| Texas Instruments Incorporated
| 24-Bit Analog-to-Digital Converters for Temperature Sensors
| Marketing part#   Voltage Range   Package-type  #pins/pkg drawing
| ADS1146IPW   2.7V - 5.25V   TSSOP   16-pin PW
| ADS1146IPWR   2.7V - 5.25V   TSSOP   16-pin PW
| ADS1147IPW   2.7V - 5.25V   TSSOP   16-pin PW
| ADS1147IPWR   2.7V - 5.25V   TSSOP   16-pin PW
| ADS1148IPW   2.7V - 5.25V   TSSOP   16-pin PW
| ADS1148IPWR   2.7V - 5.25V   TSSOP   16-pin PW
| ADS1246IPW   2.7V - 5.25V   TSSOP   16-pin PW
| ADS1246IPWR   2.7V - 5.25V   TSSOP   16-pin PW
| ADS1247IPW   2.7V - 5.25V   TSSOP   16-pin PW
| ADS1247IPWR   2.7V - 5.25V   TSSOP   16-pin PW
| ADS1248IPW   2.7V - 5.25V   TSSOP   16-pin PW
| ADS1248IPWR   2.7V - 5.25V   TSSOP   16-pin PW
[IBIS ver]   4.0
[File name]   ads1x4x.ibs
[File Rev]   1.0
[Date]   11/28/2009
[Source]   Texas Instruments Incorporated.
   Analog-eLab, HPA
   12500 TI Blvd
   Dallas, TX -75243
   For Support e-mail: elab_ibis@list.ti.com
[Notes]   Revision History
   Rev 1.0: 11/28/2009
   - Initial version of the model
   - Model based on simulations from TIspiceD
   - Model not matched to measurements
   - Ignore warnings related to ccomp, these are
   based on PVT variations as seen in simulations
[Disclaimer] This model is designed as an aid for customers of Texas Instruments.
 TI and its licensors and suppliers make no warranties, either expressed
 or implied, with respect to this  model, including the warranties of
 merchantability or fitness for a particular purpose.
 The model is provided solely on an "as is" basis. The entire risk as to
 its quality and performance is with the customer.
[Copyright] (C)Copyright 2009 Texas Instruments Incorporated.
   All rights reserved.
|   Component ADS1146PW and PWR
[Component]   ADS1146   |16-pin TSSOP PW package
[Manufacturer] TI
[Package]   |16-pin TSSOP PW and PWR package
| variable   typ   min   max
R_pkg  0.0668   0.0264   0.0907
L_pkg  2.1992nH  1.8611nH  2.5678nH
C_pkg  0.2884pF  0.2565pF  0.3511pF
[Pin] signal_name  model_name  R_pin  L_pin C_pin
   1   DVDD   POWER   0.05175  2.54903nH  0.33026pF
   2   DGND   GND   0.07117  2.04833nH  0.27033pF
   3   CLK   CLK   0.06252  1.87476nH  0.26286pF
   4   nRESET   INPUT   0.07117  2.04767nH  0.26971pF
   5   REFP   NC   0.0721   2.06639nH  0.27241pF
   6   REFN   NC   0.08688  2.36796nH  0.28566pF
   7   AINP   NC   0.06167  1.86111nH  0.25647pF
   8   AINN   NC   0.04904  2.50555nH  0.32779pF
   9   AVSS   GND   0.02642  2.28114nH  0.35109pF
   10   AVDD   POWER   0.09072  2.44998nH  0.28608pF
   11   START   INPUT   0.08853  2.40166nH  0.28835pF
   12   nCS   INPUT   0.08017  2.23009nH  0.28047pF
   13   nDRDY   OUTPUT   0.07129  2.04997nH  0.27114pF
   14   DOUT_nDRDY   DOUTPUT   0.06269  1.87807nH  0.26318pF
   15   DIN   INPUT   0.06918  2.00833nH  0.26803pF
   16   SCLK   INPUT   0.05271  2.5678nH   0.33089pF
|   Component ADS1147PW and PWR
[Component]   ADS1147   |20-pin TSSOP PW and PWR package
[Manufacturer] TI
[Package]   |20-pin TSSOP PW package
| variable   typ   min   max
R_pkg   0.0709   0.0340   0.0869
L_pkg   2.3105nH   1.5412nH   3.1530nH
C_pkg   0.3360pF   0.2711pF   0.4455pF
[Pin] signal_name  model_name  R_pin  L_pin C_pin
   1   DVDD   POWER   0.08096  3.14617nH  0.44548pF
   2   DGND   GND   0.07981  2.71014nH  0.38797pF
   3   CLK   CLK   0.06746  1.89158nH  0.27293pF
   4   nRESET   INPUT   0.06568  1.85791nH  0.27112pF
   5   REFP0_GPIO0   GPIO   0.06523  1.84931nH  0.27116pF
   6   REFN0_GPIO1   GPIO   0.07108  1.96470nH  0.27714pF
   7   VREFOUT   NC   0.03398  1.54116nH  0.30506pF
   8   VREFCOM   NC   0.07334  2.00990nH  0.28144pF
   9   AIN0_IEXC   NC   0.08690  2.85399nH  0.39588pF
   10   AIN1_IEXC   NC   0.08052  3.14616nH  0.44428pF
   11   AIN2_IEXC_GPIO2   GPIO   0.08085  3.15303nH  0.44321pF
   12   AIN3_IEXC_GPIO3   GPIO   0.08375  2.79684nH  0.38993pF
   13   AVSS   GND   0.04122  1.78526nH  0.32347pF
   14   AVDD   POWER   0.07359  2.01438nH  0.28108pF
   15   START   INPUT   0.07236  1.98988nH  0.27787pF
   16   nCS   INPUT   0.06814  1.90665nH  0.27392pF
   17   nDRDY   OUTPUT   0.06585  1.86117nH  0.27196pF
   18   DOUT_nDRDY   DOUTPUT   0.06763  1.89484nH  0.27328pF
   19   DIN   INPUT   0.07917  2.69229nH  0.38747pF
   20   SCLK   INPUT   0.08095  3.14559nH  0.44469pF
|   Component ADS1148PW and PWR
[Component]   ADS1148
[Manufacturer]  Texas Instruments Incorporated
[Package]   |28-pin TSSOP PW and PWR package
|   typ   min   max
R_pkg   0.191   0.083   0.299
L_pkg   2.756nH   1.602nH   3.911nH
C_pkg   0.569pF   0.404pF   0.734pF
[Pin] signal_name   model_name   R_pin   L_pin   C_pin
   1   DVDD   POWER   0.25840  3.78183nH   0.72612pF
   2   DGND   GND   0.25457  3.37203nH   0.65437pF
   3   CLK   CLK   0.27139  2.95777nH   0.47887pF
   4   nRESET   INPUT   0.24262  2.60943nH   0.42484pF
   5   REFP0_GPIO0   GPIO   0.23670  2.55749nH   0.43312pF
   6   REFN0_GPIO1   GPIO   0.19699  2.23854nH   0.41962pF
   7   REFP1   NC   0.16925  2.01926nH   0.40844pF
   8   REFN1   NC   0.15863  1.93718nH   0.40408pF
   9   VREFOUT   NC   0.08283  1.60169nH   0.43637pF
   10   VREFCOM   NC   0.18323  2.13341nH   0.41480pF
   11   AIN0_IEXC   NC   0.21768  2.41321nH   0.41552pF
   12   AIN1_IEXC   NC   0.27481  2.99152nH   0.47926pF
   13   AIN4_IEXC_GPIO4   GPIO   0.26374  3.45284nH   0.65872pF
   14   AIN5_IEXC_GPIO5   GPIO   0.26014  3.80161nH   0.72855pF
   15   AIN6_IEXC_GPIO6   GPIO   0.27369  3.91108nH   0.73394pF
   16   AIN7_IEXC_GPIO7   GPIO   0.28429  3.61685nH   0.66751pF
   17   AIN2_IEXC_GPIO2   GPIO   0.29927  3.19031nH   0.48711pF
   18   AIN3_IEXC_GPIO3   GPIO   0.21114  2.36074nH   0.41327pF
   19   IEXC2   NC   0.17260  2.04890nH   0.41119pF
   20   IEXC1   NC   0.15867  1.93751nH   0.40587pF
   21   AVSS   GND   0.08769  1.65289nH   0.44333pF
   22   AVDD   POWER   0.19052  2.18715nH   0.41522pF
   23   START   INPUT   0.19562  2.22790nH   0.41629pF
   24   nCS   INPUT   0.21539  2.38631nH   0.42471pF
   25   nDRDY   OUTPUT   0.24299  2.61259nH   0.42589pF
   26   DOUT_nDRDY   DOUTPUT   0.27156  2.95896nH   0.47947pF
   27   DIN   INPUT   0.25335  3.35997nH   0.65372pF
   28   SCLK   INPUT   0.25851  3.78132nH   0.72511pF
|   Component ADS1246PW and PWR
[Component]   ADS1246   |16-pin TSSOP PW package
[Manufacturer] TI
[Package]   |16-pin TSSOP PW and PWR package
| variable   typ   min   max
R_pkg  0.0668   0.0264   0.0907
L_pkg  2.1992nH  1.8611nH  2.5678nH
C_pkg  0.2884pF  0.2565pF  0.3511pF
[Pin] signal_name  model_name  R_pin  L_pin C_pin
   1   DVDD   POWER   0.05175  2.54903nH  0.33026pF
   2   DGND   GND   0.07117  2.04833nH  0.27033pF
   3   CLK   CLK   0.06252  1.87476nH  0.26286pF
   4   nRESET   INPUT   0.07117  2.04767nH  0.26971pF
   5   REFP   NC   0.0721   2.06639nH  0.27241pF
   6   REFN   NC   0.08688  2.36796nH  0.28566pF
   7   AINP   NC   0.06167  1.86111nH  0.25647pF
   8   AINN   NC   0.04904  2.50555nH  0.32779pF
   9   AVSS   GND   0.02642  2.28114nH  0.35109pF
   10   AVDD   POWER   0.09072  2.44998nH  0.28608pF
   11   START   INPUT   0.08853  2.40166nH  0.28835pF
   12   nCS   INPUT   0.08017  2.23009nH  0.28047pF
   13   nDRDY   OUTPUT   0.07129  2.04997nH  0.27114pF
   14   DOUT_nDRDY   DOUTPUT   0.06269  1.87807nH  0.26318pF
   15   DIN   INPUT   0.06918  2.00833nH  0.26803pF
   16   SCLK   INPUT   0.05271  2.5678nH   0.33089pF
|   Component ADS1247PW and PWR
[Component]   ADS1247   |20-pin TSSOP PW and PWR package
[Manufacturer] TI
[Package]   |20-pin TSSOP PW package
| variable   typ   min   max
R_pkg   0.0709   0.0340   0.0869
L_pkg   2.3105nH   1.5412nH   3.1530nH
C_pkg   0.3360pF   0.2711pF   0.4455pF
[Pin] signal_name  model_name  R_pin  L_pin C_pin
   1   DVDD   POWER   0.08096  3.14617nH  0.44548pF
   2   DGND   GND   0.07981  2.71014nH  0.38797pF
   3   CLK   CLK   0.06746  1.89158nH  0.27293pF
   4   nRESET   INPUT   0.06568  1.85791nH  0.27112pF
   5   REFP0_GPIO0   GPIO   0.06523  1.84931nH  0.27116pF
   6   REFN0_GPIO1   GPIO   0.07108  1.96470nH  0.27714pF
   7   VREFOUT   NC   0.03398  1.54116nH  0.30506pF
   8   VREFCOM   NC   0.07334  2.00990nH  0.28144pF
   9   AIN0_IEXC   NC   0.08690  2.85399nH  0.39588pF
   10   AIN1_IEXC   NC   0.08052  3.14616nH  0.44428pF
   11   AIN2_IEXC_GPIO2   GPIO   0.08085  3.15303nH  0.44321pF
   12   AIN3_IEXC_GPIO3   GPIO   0.08375  2.79684nH  0.38993pF
   13   AVSS   GND   0.04122  1.78526nH  0.32347pF
   14   AVDD   POWER   0.07359  2.01438nH  0.28108pF
   15   START   INPUT   0.07236  1.98988nH  0.27787pF
   16   nCS   INPUT   0.06814  1.90665nH  0.27392pF
   17   nDRDY   OUTPUT   0.06585  1.86117nH  0.27196pF
   18   DOUT_nDRDY   DOUTPUT   0.06763  1.89484nH  0.27328pF
   19   DIN   INPUT   0.07917  2.69229nH  0.38747pF
   20   SCLK   INPUT   0.08095  3.14559nH  0.44469pF
|   Component ADS1248PW and PWR
[Component]   ADS1248
[Manufacturer]  Texas Instruments Incorporated
[Package]   |28-pin TSSOP PW and PWR package
|   typ   min   max
R_pkg   0.191   0.083   0.299
L_pkg   2.756nH   1.602nH   3.911nH
C_pkg   0.569pF   0.404pF   0.734pF
[Pin] signal_name   model_name   R_pin   L_pin   C_pin
   1   DVDD   POWER   0.25840  3.78183nH   0.72612pF
   2   DGND   GND   0.25457  3.37203nH   0.65437pF
   3   CLK   CLK   0.27139  2.95777nH   0.47887pF
   4   nRESET   INPUT   0.24262  2.60943nH   0.42484pF
   5   REFP0_GPIO0   GPIO   0.23670  2.55749nH   0.43312pF
   6   REFN0_GPIO1   GPIO   0.19699  2.23854nH   0.41962pF
   7   REFP1   NC   0.16925  2.01926nH   0.40844pF
   8   REFN1   NC   0.15863  1.93718nH   0.40408pF
   9   VREFOUT   NC   0.08283  1.60169nH   0.43637pF
   10   VREFCOM   NC   0.18323  2.13341nH   0.41480pF
   11   AIN0_IEXC   NC   0.21768  2.41321nH   0.41552pF
   12   AIN1_IEXC   NC   0.27481  2.99152nH   0.47926pF
   13   AIN4_IEXC_GPIO4   GPIO   0.26374  3.45284nH   0.65872pF
   14   AIN5_IEXC_GPIO5   GPIO   0.26014  3.80161nH   0.72855pF
   15   AIN6_IEXC_GPIO6   GPIO   0.27369  3.91108nH   0.73394pF
   16   AIN7_IEXC_GPIO7   GPIO   0.28429  3.61685nH   0.66751pF
   17   AIN2_IEXC_GPIO2   GPIO   0.29927  3.19031nH   0.48711pF
   18   AIN3_IEXC_GPIO3   GPIO   0.21114  2.36074nH   0.41327pF
   19   IEXC2   NC   0.17260  2.04890nH   0.41119pF
   20   IEXC1   NC   0.15867  1.93751nH   0.40587pF
   21   AVSS   GND   0.08769  1.65289nH   0.44333pF
   22   AVDD   POWER   0.19052  2.18715nH   0.41522pF
   23   START   INPUT   0.19562  2.22790nH   0.41629pF
   24   nCS   INPUT   0.21539  2.38631nH   0.42471pF
   25   nDRDY   OUTPUT   0.24299  2.61259nH   0.42589pF
   26   DOUT_nDRDY   DOUTPUT   0.27156  2.95896nH   0.47947pF
   27   DIN   INPUT   0.25335  3.35997nH   0.65372pF
   28   SCLK   INPUT   0.25851  3.78132nH   0.72511pF
|   Model Selectors
[Model Selector]   INPUT
IN_3   2.70V - 3.30V Input Model
IN_5   4.75V - 5.25V Input Model
[Model Selector]   CLK
CLK_3   2.70V - 3.30V Clk Model
CLK_5   4.75V - 5.25V Clk Model
[Model Selector]   OUTPUT
OUT_3   2.70V - 3.30V Output Model
OUT_5   4.75V - 5.25V Output Model
[Model Selector]   DOUTPUT
DOUT_3   2.70V - 3.30V DOutput Model
DOUT_5   4.75V - 5.25V DOutput Model
[Model Selector]   GPIO
GPIO_3   2.70V - 3.30V GPIO Model
GPIO_5   4.75V - 5.25V GPIO Model
| Models and submodels in the file (10): OUT_3 (Output), OUT_5 (Output), DOUT_3 (3-state), DOUT_5 (3-state), IN_3 (Input), IN_5 (Input), CLK_3 (Input), CLK_5 (Input), GPIO_3 (I/O), GPIO_5 (I/O)
